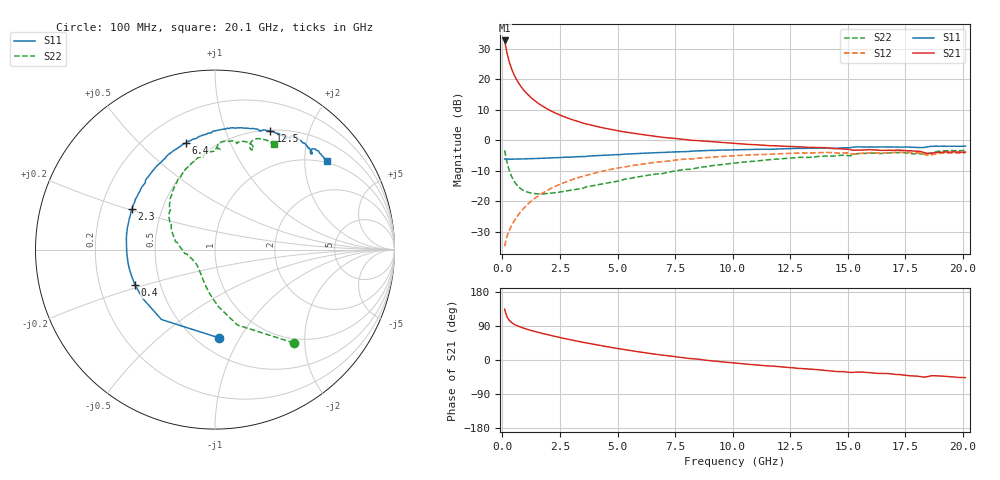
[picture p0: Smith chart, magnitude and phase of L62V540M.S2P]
!  Infineon Technologies AG
! BFR380L3 , PF131585-7, No.6, Th 09.10.01, soldered on pcb-board, measured with PP GSG850
!  Vce=2.5 V,  Ic=40.0 mA
! Common Emitter S-Parameters:  15. November 2001
#  GHz  S  MA  R  50
! f  S11  S21  S12  S22
! GHz  Mag  Ang  Mag  Ang  Mag  Ang  Mag  Ang
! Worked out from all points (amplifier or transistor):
!   201 points, 100 MHz to 20.1 GHz, reference 50 ohm
!   highest |S21| = 32.7 dB at 100 MHz (marker M1)
!   |S21| within 3 dB of that: start of sweep to 175.3 MHz
!   unconditionally stable (mu >= 1): 991.9 MHz to 4.347 GHz
!   at 3.4 GHz: K = 1.02, MAG = 8.2 dB, |S12| = -12.1 dB
!   at 10.1 GHz: K = 0.96, MSG = 2.0 dB, |S12| = -5.1 dB
!   at 20.1 GHz: K = 0.99, MSG = 0.1 dB, |S12| = -4.2 dB
!   S11 on the Smith chart (normalised r, x): 100 MHz: 0.63, -0.82; 400 MHz: 0.36, -0.19; 2.3 GHz: 0.34, +0.21; 6.4 GHz: 0.36, +0.70; 12.5 GHz: 0.51, +1.44; 20.1 GHz: 0.94, +2.55
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0.1  0.4911 -87.7  43.32 134.0  0.01818 61.4  0.6802 -49.8
0.2  0.4906 -127.4  27.38 114.2  0.02644 57.9  0.439 -73.3
0.3  0.4858 -145.6  19.42 104.8  0.03295 59.0  0.3198 -86.4
0.4  0.4874 -155.9  14.93 99.0  0.03937 61.6  0.2546 -95.6
0.5  0.4874 -162.8  12.09 94.8  0.04594 63.9  0.2153 -102.9
0.6  0.4897 -168.0  10.14 91.7  0.05283 65.4  0.1897 -109.0
0.7  0.4902 -172.4  8.749 89.0  0.05976 66.7  0.1721 -114.4
0.8  0.4903 -175.8  7.684 86.6  0.06696 67.5  0.1598 -119.1
1  0.4929 178.5  6.188 82.5  0.08113 68.3  0.1444 -127.0
1.2  0.497 173.6  5.185 78.8  0.09574 68.5  0.1367 -133.5
1.5  0.5017 167.5  4.181 73.8  0.1173 67.9  0.1315 -141.3
1.9  0.5077 160.4  3.338 67.8  0.146 66.1  0.1322 -149.7
2.3  0.5144 154.1  2.791 62.2  0.1744 64.0  0.1373 -156.8
3.5  0.5377 136.8  1.909 46.7  0.2563 56.1  0.1616 -171.8
4.8  0.5729 121.6  1.48 32.3  0.336 47.0  0.206 171.8
6.4  0.6169 105.4  1.19 17.3  0.4215 35.6  0.2689 154.6
6.8  0.626 101.7  1.137 13.8  0.4402 32.6  0.2807 150.2
10.1  0.6957 77.6  0.8808 -8.1  0.5549 10.9  0.4215 121.9
12.5  0.7279 65.1  0.7872 -20.2  0.6077 -3.6  0.5077 102.9
13.5  0.7348 60.5  0.7618 -24.6  0.6176 -9.4  0.5311 96.5
16.8  0.7713 48.2  0.6836 -36.1  0.6245 -25.1  0.6195 76.5
20.1  0.7957 38.5  0.6387 -46.6  0.6189 -38.6  0.6755 60.9
